| Texas Instruments Incorporated
| Digital PWM System Controller
| Marketing part#   Voltage Range   Package-type   #pins/pkg drawing
| UCD9240RGCR   3.0V - 3.6V   QFN   64-pin
| UCD9240RGCT   3.0V - 3.6V   QFN   64-pin
| UCD9240PFCR   3.0V - 3.6V   QFP   80-pin
| UCD9240PFCT   3.0V - 3.6V   QFP   80-pin
[IBIS ver]   4.0
[File name]   ucd9240.ibs
[File Rev]   1.1
[Date]   09/29/2010
[Source]   Simulations in SPECTRE
   Texas Instruments Incorporated.
   Analog-eLab, HPA
   12500 TI Blvd
   Dallas, TX -75243
   For Support e-mail: elab_ibis@list.ti.com
[Notes]   Revision History
   Rev 1.0: 01/05/2010
   - Initial version of the model
   - Model based on simulations from Spectre
   - Model not matched to measurements
   - Ignore warnings related to ccomp, these are
   based on PVT conditions as seen in simulations
   - Non-monotonic behavior is as per buffer simulations
   Rev 1.1: 09/29/2010
   - Added package model for 80-pin QFP package
   - Eliminated ccomp warnings by numerically arranging ccomp
   - 64-pin [component/pkg was incorrectly named *PFC, now
   corrected to *RGC
   - non-monotonic warnings still related to buffer behavior
   seen in simulations
[Disclaimer] This model is designed as an aid for customers of Texas Instruments.
 TI and its licensors and suppliers make no warranties, either expressed
 or implied, with respect to this  model, including the warranties of
 merchantability or fitness for a particular purpose.
 The model is provided solely on an "as is" basis. The entire risk as to
 its quality and performance is with the customer.
[Copyright] (C)Copyright 2010 Texas Instruments Incorporated.
   All rights reserved.
|   Component UCD940RGC
[Component]   UCD9240RGC
[Manufacturer]  Texas Instruments Incorporated
[Package]   |64-pin QFN package
|   typ   min   max
R_pkg   0.1178   0.0994   0.1361
L_pkg   2.6934nH   2.2542nH   3.1326nH
C_pkg   0.3299pF   0.2790pF   0.3808pF
[Pin] signal_name   model_name   R_pin   L_pin   C_pin
   1   CS4A   TERM   0.13609  3.13264nH   0.34764pF
   2   CS3A   TERM   0.12598  2.88745nH   0.37020pF
   3   CS2A   TERM   0.11801  2.70820nH   0.35698pF
   4   VIN_IIN   TERM   0.11243  2.57494nH   0.34578pF
   5   VTRACK   TERM   0.10937  2.52081nH   0.34125pF
   6   TEMP   TERM   0.10828  2.46541nH   0.31963pF
   7   V33DIO1   POWER   0.10863  2.45321nH   0.30672pF
   8   DVSS1   GND   0.10985  2.46569nH   0.29065pF
   9   NRESET   TERM   0.10853  2.43935nH   0.29142pF
   10   TRCK   TERM   0.10888  2.45722nH   0.30499pF
   11   FAULT1A   TERM   0.10945  2.48954nH   0.31724pF
   12   FAULT1B   TERM   0.11198  2.55496nH   0.33589pF
   13   FAULT2A   TERM   0.11460  2.64095nH   0.35271pF
   14   FAULT2B   TERM   0.12122  2.77218nH   0.35779pF
   15   PMBUSCLK   IO   0.12692  2.90716nH   0.36485pF
   16   PMBUSDATA   IO   0.13564  3.12442nH   0.34751pF
   17   DPWM1A   TERM   0.13092  3.02659nH   0.33670pF
   18   DPWM1B   TERM   0.11565  2.67718nH   0.34805pF
   19   DPWM2A   TERM   0.10908  2.52402nH   0.34137pF
   20   DPWM2B   TERM   0.10434  2.40588nH   0.33254pF
   21   DPWM3A   TERM   0.10120  2.34876nH   0.32797pF
   22   SRE1A   TERM   0.09981  2.28965nH   0.30393pF
   23   DPWM4A   TERM   0.09943  2.26332nH   0.29099pF
   24   SRE1B   TERM   0.09979  2.25793nH   0.28322pF
   25   FAULT3A   TERM   0.10082  2.27762nH   0.27901pF
   26   DVSS2   GND   0.05012  1.90467nH   0.33013pF
   27   PMBUSALERT   TERM   0.09967  2.28695nH   0.30950pF
   28   PMBUSCTRL   TERM   0.10131  2.33100nH   0.32681pF
   29   SRE3A   TERM   0.10557  2.44923nH   0.34754pF
   30   SRE4A   TERM   0.11253  2.58741nH   0.35253pF
   31   TMUX0   TERM   0.12145  2.78670nH   0.36722pF
   32   TMUX1   TERM   0.13307  3.06270nH   0.34634pF
   33   SRE2A   TERM   0.13073  3.01550nH   0.33729pF
   34   FAULT4A   TERM   0.12266  2.80961nH   0.36052pF
   35   SRE2B   TERM   0.11638  2.66234nH   0.34862pF
   36   FANTACH_TCK  TERM   0.11286  2.56883nH   0.34340pF
   37   SYNCOUT_TDO  TERM   0.10950  2.50747nH   0.33811pF
   38   SYNCIN_TDI   TERM   0.10875  2.46130nH   0.31582pF
   39   POWERGOOD_TMS   TERM   0.10838  2.43555nH   0.30240pF
   40   NTRST   TERM   0.10871  2.42987nH   0.28408pF
   41   FANPWM   TERM   0.10956  2.44664nH   0.28799pF
   42   TMUX2   TERM   0.10857  2.43804nH   0.30731pF
   43   DVSS3   GND   0.05454  2.06658nH   0.36989pF
   44   V33DIO2   POWER   0.10874  2.47438nH   0.33463pF
   45   V33D   POWER   0.11065  2.54664nH   0.34854pF
   46   V33A   POWER   0.11512  2.63652nH   0.35492pF
   47   V33DIO2   POWER   0.06101  2.34670nH   0.42070pF
   48   AVSS2   GND   0.12928  2.98599nH   0.34291pF
   49   AVSS1   GND   0.06956  2.74533nH   0.40404pF
   50   EAP1   TERM   0.12795  2.91571nH   0.38083pF
   51   EAN1   TERM   0.11782  2.69249nH   0.36069pF
   52   EAP2   TERM   0.10988  2.51176nH   0.34570pF
   53   EAN2   TERM   0.10446  2.41048nH   0.33724pF
   54   EAP3   TERM   0.10133  2.31804nH   0.31105pF
   55   EAN3   TERM   0.09979  2.26987nH   0.29630pF
   56   EAP4   TERM   0.09958  2.25421nH   0.28769pF
   57   EAN4   TERM   0.10052  2.27347nH   0.28486pF
   58   V33FB   POWER   0.10117  2.29789nH   0.28501pF
   59   CS1A   TERM   0.09944  2.28345nH   0.29939pF
   60   ADDRSENS1   TERM   0.10087  2.32459nH   0.32533pF
   61   ADDRSENS0   TERM   0.10459  2.43370nH   0.34487pF
   62   CS2B   TERM   0.11090  2.56040nH   0.35002pF
   63   CS1B   TERM   0.11965  2.75738nH   0.36780pF
   64   AVSS3   GND   0.06507  2.57083nH   0.39061pF
|   Component UCD940PFC
[Component]   UCD9240PFC
[Manufacturer]  Texas Instruments Incorporated
[Package]   |80-pin QFP package
|   typ   min   max
R_pkg   0.0998   0.0910   0.1122
L_pkg   5.1178nH   4.5739nH   6.0875nH
C_pkg   0.7737pF   0.6543pF   1.0508pF
[Pin] signal_name   model_name   R_pin   L_pin   C_pin
   1   ADCref   TERM   0.10949  5.61973nH   0.71383pF
   2   CS4A   TERM   0.10597  5.40633nH   0.82858pF
   3   CS3A   TERM   0.10332  5.25836nH   0.81119pF
   4   CS2A   TERM   0.10143  5.12685nH   0.79041pF
   5   VinIin   TERM   0.10023  5.02455nH   0.77170pF
   6   VTRACK   TERM   0.09965  4.96064nH   0.69642pF
   7   Temp   TERM   0.09947  4.83733nH   0.69166pF
   8   V33DIO   POWER   0.09994  4.76450nH   0.74233pF
   9   DVss   GND   0.05485  5.84527nH   1.09380pF
   10   DiagLED   TERM   0.10157  4.78301nH   0.67177pF
   11   SRE1B   TERM   0.10253  4.80357nH   0.66641pF
   12   SRE1A   TERM   0.10354  6.08752nH   1.04824pF
   13   nRESET   TERM   0.10232  4.81534nH   0.74437pF
   14   TRCK   TERM   0.10365  4.92640nH   0.69381pF
   15   FAULT1A   TERM   0.10361  5.04538nH   0.69830pF
   16   FAULT1B   TERM   0.10568  5.14146nH   0.77587pF
   17   FAULT2A   TERM   0.10581  5.22184nH   0.79310pF
   18   FAULT2B   TERM   0.10887  5.37885nH   0.81554pF
   19   PMBus_Clk   IO   0.10958  5.48681nH   0.82589pF
   20   PMBus_Data   IO   0.11220  5.68248nH   0.71565pF
   21   dPWM1A   TERM   0.10837  5.61223nH   0.70610pF
   22   dPWM1B   TERM   0.09824  5.25940nH   0.81086pF
   23   dPWM2A   TERM   0.09657  5.13072nH   0.79867pF
   24   dPWM2B   TERM   0.09535  5.01195nH   0.77940pF
   25   dPWM3A   TERM   0.09405  4.90666nH   0.76065pF
   26   dPWM3B   TERM   0.09324  4.83636nH   0.68363pF
   27   dPWM4A   TERM   0.09255  4.69712nH   0.67717pF
   28   dPWM4B   TERM   0.09224  4.60837nH   0.72712pF
   29   FAULT3A   TERM   0.09363  5.88478nH   1.03795pF
   30   SYNCOUT   TERM   0.09232  4.59525nH   0.65425pF
   31   SYNCIN   TERM   0.09199  4.58884nH   0.65701pF
   32   FANTACH   TERM   0.09304  5.87320nH   1.04454pF
   33   SRE4A   TERM   0.09181  4.60044nH   0.73472pF
   34   DVss   GND   0.04922  4.51271nH   0.71909pF
   35   PMBus_Alert  TERM   0.09285  4.82507nH   0.68882pF
   36   PMBus_Cntrl  TERM   0.09426  4.90652nH   0.76577pF
   37   SRE2B   TERM   0.09678  5.03635nH   0.78834pF
   38   SRE3A   TERM   0.10010  5.19766nH   0.81041pF
   39   TMUX0   TERM   0.10372  5.36609nH   0.82970pF
   40   TMUX1   TERM   0.10879  5.61195nH   0.71639pF
   41   FAULT3B   TERM   0.10790  5.59213nH   0.70761pF
   42   FAULT4A   TERM   0.10568  5.40500nH   0.82185pF
   43   FAULT4B   TERM   0.10400  5.27653nH   0.80372pF
   44   TCK   TERM   0.10382  5.17997nH   0.78944pF
   45   TDO   TERM   0.10190  5.06190nH   0.76988pF
   46   TDI   TERM   0.10211  5.01384nH   0.69573pF
   47   TMS   TERM   0.10089  4.86815nH   0.68915pF
   48   nTRST   TERM   0.10130  4.79358nH   0.74019pF
   49   POWERGOOD   TERM   0.10240  6.06314nH   1.05080pF
   50   SRE4B   TERM   0.10147  4.78099nH   0.66450pF
   51   SRE2A   TERM   0.10115  4.77345nH   0.66395pF
   52   SRE3B   TERM   0.10199  6.05141nH   1.05031pF
   53   FANPWM   TERM   0.10023  4.76791nH   0.74122pF
   54   TMUX2   TERM   0.10007  4.84638nH   0.69082pF
   55   DVss   GND   0.05344  4.77326nH   0.73623pF
   56   V33DIO   POWER   0.10063  5.03300nH   0.76983pF
   57   V33D   POWER   0.10113  5.12098nH   0.78602pF
   58   V33A   POWER   0.10275  5.24682nH   0.81005pF
   59   BPCap   TERM   0.05559  5.17106nH   0.86605pF
   60   AVss   GND   0.10667  5.56132nH   0.71258pF
   61   AVss   GND   0.06024  5.53090nH   0.75367pF
   62   EAp1   TERM   0.11009  5.49113nH   0.84149pF
   63   EAn1   TERM   0.10564  5.30494nH   0.81949pF
   64   EAp2   TERM   0.10192  5.13466nH   0.79508pF
   65   EAn2   TERM   0.09887  4.99333nH   0.77299pF
   66   EAp3   TERM   0.09644  4.89061nH   0.69435pF
   67   EAn3   TERM   0.09435  4.69658nH   0.68223pF
   68   EAp4   TERM   0.09313  4.59917nH   0.72630pF
   69   EAn4   TERM   0.09385  5.86214nH   1.03100pF
   70   V33FB   POWER   0.09299  4.59368nH   0.65077pF
   71   AD14   TERM   0.09224  4.58450nH   0.65636pF
   72   AD13   TERM   0.09282  5.85838nH   1.04227pF
   73   CS4B   TERM   0.09102  4.57390nH   0.73080pF
   74   CS3B   TERM   0.09121  4.66046nH   0.68059pF
   75   CS1A   TERM   0.09211  4.79485nH   0.68802pF
   76   AddrSens1   TERM   0.09349  4.87107nH   0.76518pF
   77   AddrSens0   TERM   0.09555  4.98663nH   0.78376pF
   78   CS2B   TERM   0.09834  5.13332nH   0.80445pF
   79   CS1B   TERM   0.10188  5.29553nH   0.82337pF
   80   AVss   GND   0.05600  5.34286nH   0.73872pF
[Model] TERM
Model_type Terminator
C_comp   0  0  0
| variable   typ   min   max
[Voltage Range]   3.30000V  3.00000V  3.60000V
[POWER Clamp Reference]  3.30000V  3.00000V  3.60000V
[GND Clamp Reference]   0.00000V  0.00000V  0.00000V
[Temperature Range]   27   110   -40
| Models and submodels in the file (2): TERM (Terminator), IO (I/O)
